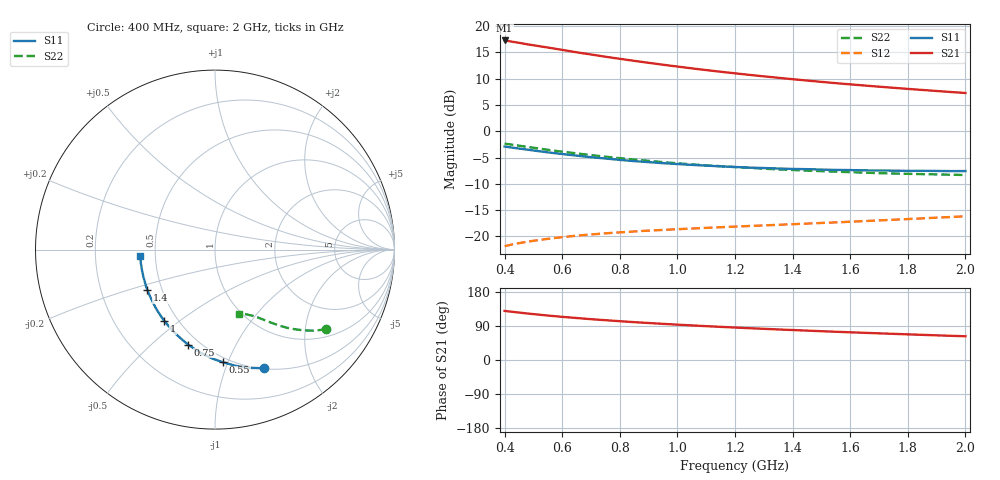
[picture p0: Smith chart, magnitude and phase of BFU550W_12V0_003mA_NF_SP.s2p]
! Filename:  P:\Prog\Test\Noise\ATS_data\Testdata_Net\06 Compressed Noise after Statistics\BFU550W_APM2013_11_D05_12p0V_003mA_NF_CM01_D.sf
! Date/Time: Tue 26/Mar/2013 16:25:25
! BFU550W_APM2013_11_D05_12p0V_1to35mA_NF_CM01_Bias3_R.sf
! Noise Parameter Data File
! BFU550W_APM2013_11_D05_12p0V_1to35mA_NF_CM01
! Date/time: Mon Mar 25 15:58:35 2013
! VAR V_out= 12.001000
! VAR I_out= 2.995000
! VAR V_in= 0.790700
! VAR I_in= 0.023905
! Device data file deembeded for feedlines and parallel
! Original file: \06 Compressed Noise after Statistics\BFU550W_APM2013_11_D05_12p0V_003mA_NF_CM01_R.sf
! Feed-files: PR019V01_070313_Feed1.s2p, PR019V01_070313_Feed2.s2p
! Parallel-file: PR019V01_070313_Par.s2p
# MHz S MA R 50
!  Freq-MHz  S11-mag  S11-arg  S21-mag  S21-arg  S12-mag  S12-arg  S22-mag  S22-arg
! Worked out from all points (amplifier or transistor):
!   37 points, 400 MHz to 2 GHz, reference 50 ohm
!   highest |S21| = 17.2 dB at 400 MHz (marker M1)
!   |S21| within 3 dB of that: start of sweep to 739.5 MHz
!   unconditionally stable (mu >= 1): nowhere
!   at 500 MHz: K = 0.37, MSG = 18.6 dB, |S12| = -20.8 dB
!   at 1.1 GHz: K = 0.72, MSG = 15.0 dB, |S12| = -18.4 dB
!   at 2 GHz: K = 1.00, MSG = 11.7 dB, |S12| = -16.2 dB
!   lowest NFmin = 0.54 dB at 420 MHz
!   S11 on the Smith chart (normalised r, x): 400 MHz: 0.51, -1.37; 550 MHz: 0.46, -0.96; 750 MHz: 0.44, -0.66; 1 GHz: 0.42, -0.44; 1.4 GHz: 0.42, -0.23; 2 GHz: 0.41, -0.03
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400  0.7146 -67.5  7.269 129.5  0.08093 55.7  0.761 -35.5
420  0.7015 -70.2  7.122 127.7  0.08328 54.7  0.7479 -36.6
440  0.69 -72.8  6.976 126.0  0.08544 53.7  0.7347 -37.6
480  0.6674 -77.7  6.672 122.7  0.08928 52.1  0.7085 -39.5
500  0.6558 -80.3  6.544 121.1  0.09106 51.3  0.6959 -40.4
550  0.6292 -86.0  6.226 117.3  0.09498 49.7  0.6654 -42.5
600  0.6068 -91.5  5.918 113.9  0.09856 48.2  0.6383 -44.2
650  0.5861 -96.4  5.61 110.8  0.1018 47.1  0.6154 -45.8
700  0.5662 -101.3  5.351 107.7  0.1045 46.1  0.5923 -47.4
750  0.5503 -105.8  5.093 105.0  0.1071 45.4  0.5726 -48.6
800  0.5336 -110.1  4.867 102.4  0.1094 44.8  0.5542 -49.8
850  0.5197 -114.3  4.654 99.9  0.1116 44.3  0.5372 -50.8
950  0.4967 -121.8  4.277 95.4  0.1155 43.7  0.5081 -52.8
1000  0.4872 -125.5  4.107 93.3  0.1173 43.5  0.4958 -53.6
1100  0.4706 -132.0  3.804 89.3  0.1207 43.6  0.4737 -55.4
1200  0.4571 -138.2  3.544 85.7  0.1241 43.7  0.4561 -57.0
1300  0.4467 -143.9  3.315 82.3  0.1274 44.2  0.4408 -58.4
1400  0.438 -149.3  3.117 79.1  0.1308 44.8  0.4281 -59.9
1500  0.432 -154.2  2.94 76.0  0.1344 45.4  0.4175 -61.4
1600  0.4273 -159.0  2.784 73.1  0.1381 46.2  0.4081 -62.9
1750  0.422 -165.4  2.583 69.0  0.1442 47.6  0.3962 -65.1
2000  0.4182 -175.3  2.305 62.6  0.1557 49.7  0.3836 -69.2
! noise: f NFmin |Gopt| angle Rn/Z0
400  0.5453  0.3347  33.14  0.1413
460  0.5578  0.3326  39.5  0.1351
600  0.6195  0.3354  43.99  0.145
800  0.6511  0.3344  66.35  0.1214
1000  0.6834  0.3501  78.81  0.1214
1200  0.7586  0.3516  93.87  0.1083
1400  0.8367  0.3584  109.3  0.0857
1600  0.7996  0.352  125.5  0.0809
1800  0.9241  0.37  139.5  0.0716
2000  0.9634  0.3699  154.4  0.0675
